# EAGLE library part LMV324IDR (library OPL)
General purpose LOW Voltage, Rail-to-Rail Output Amplifiers http://www.fairchildsemi.com/ds/LM/LMV358.pdf
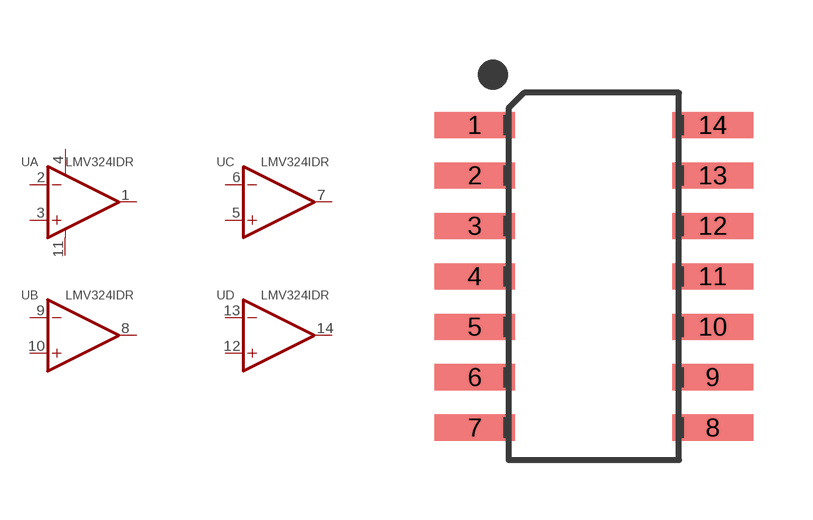
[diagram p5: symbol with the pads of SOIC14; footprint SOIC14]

Designator prefix U; gates A=OP-AMP+- B=OP-AMP C=OP-AMP D=OP-AMP

## LMV324IDR-1100030P1  [SOIC14]
1  A:OUT  out
2  A:IN-  in
3  A:IN+  in
4  A:V+  pwr
5  C:IN+  in
6  C:IN-  in
7  C:OUT  out
8  B:OUT  out
9  B:IN-  in
10  B:IN+  in
11  A:V-  pwr
12  D:IN+  in
13  D:IN-  in
14  D:OUT  out

## Footprint SOIC14 (pad centres in mm)
smd 2.032 x 0.66: 1 -2.997,3.81; 2 -2.997,2.54; 3 -2.997,1.27; 4 -2.997,0; 5 -2.997,-1.27; 6 -2.997,-2.54; 7 -2.997,-3.81; 8 2.997,-3.81; 9 2.997,-2.54; 10 2.997,-1.27; 11 2.997,0; 12 2.997,1.27; 13 2.997,2.54; 14 2.997,3.81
